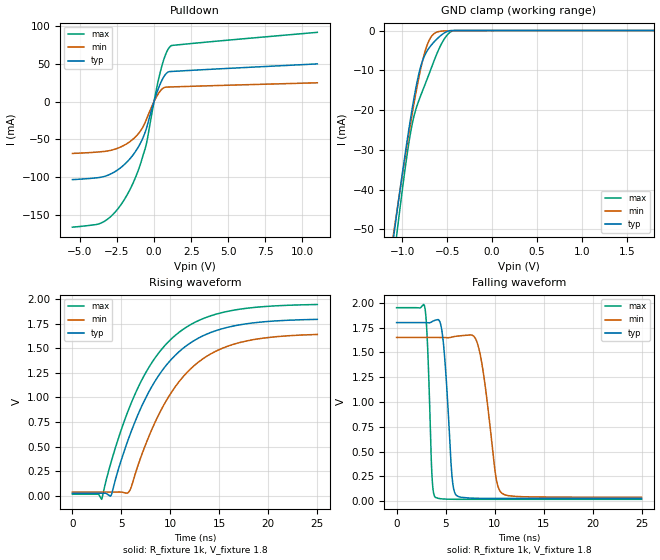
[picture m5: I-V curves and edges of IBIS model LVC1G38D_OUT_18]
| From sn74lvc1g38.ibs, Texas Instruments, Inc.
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[Model]   LVC1G38D_OUT_18
Model_type  Open_drain
Enable   Active-High
Vref =   1.8
Rref =   1000
Cref =   30p
Vmeas =   0.9
| variable   typ   min   max
C_comp   4.16pF   3.36pF   5.08pF
| C_pulldown   8.66pF   4.89pF   13.94pF
| C_tri-state   4.16pF   3.36pF   5.08pF
[Temperature Range]   40   100   -40
| Ambient temperature   25   85   -40
[Voltage range]   1.8   1.65   1.95
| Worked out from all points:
|   slope of the pulldown table from 0 to 0.27 V, typ, clamps not added: 16.8 ohm
|   GND clamp passes 1 mA (typ) near -0.56 V on its own axis
|   rising waveform, R_fixture 1k, V_fixture 1.8: 20-80 % time 5.58ns typ, 5.52ns min, 5.61ns max; typ from 0.027 V to 1.79 V
|   falling waveform, R_fixture 1k, V_fixture 1.8: 20-80 % time 650ps typ, 1.18ns min, 384ps max; typ from 1.8 V to 0.027 V
[GND Clamp]
| LVC1G38D_OUT_18
|   Voltage   I(typ)   I(min)   I(max)
-5.5V     -916.4mA   -845.5mA   -1.045A
-1.115V   -54.98mA   -53.86mA   -61.45mA
-1.085V   -49.92mA   -49.21mA   -55.72mA
-1.055V   -44.94mA   -44.63mA   -50.09mA
-910mV    -22.43mA   -23.64mA   -25.96mA
-860mV    -15.79mA   -17.12mA   -20.67mA
-795mV    -9.083mA   -9.641mA   -16.36mA
-725mV    -5.18mA    -3.758mA   -12.29mA
-670mV    -3.475mA   -1.333mA   -9.01mA
-565mV    -1.144mA   -165.1uA   -3.4mA
-475mV    -48.31uA   -65.08uA   -556uA
1.8V      20.21pA    264.6pA    784.5pA
[Pulldown]
| LVC1G38D_OUT_18
|   Voltage   I(typ)   I(min)   I(max)
-5.5V     -103.4mA   -68.72mA   -166.4mA
-3.32V    -99.02mA   -66.01mA   -158.4mA
-2.515V   -91.42mA   -62.29mA   -144mA
-1.745V   -78.46mA   -54.7mA    -121.2mA
-1.13V    -62.51mA   -44.26mA   -94.65mA
-600mV    -40.65mA   -27.77mA   -62.5mA
-450mV    -31.26mA   -20.5mA    -49.8mA
10mV      654.1uA    412.9uA    1.064mA
410mV     23.11mA    13.75mA    38.36mA
775mV     36.12mA    19.1mA     62.15mA
1.11V     39.81mA    19.36mA    73.37mA
11V       49.91mA    24.89mA    91.75mA
[Ramp]
| LVC1G38D_OUT_18
| variable   typ   min   max
dV/dt_r   1.08/5.59E-09   0.97/5.53E-09   1.19/5.63E-09
dV/dt_f   1.08/6.67E-10   0.98/1.20E-09   1.18/3.96E-10
R_load = 1k
[Rising Waveform]
| LVC1G38D_OUT_18
R_fixture =   1k
C_fixture =   0
L_fixture =   0
V_fixture =   1.8
V_fixture_min = 1.65
V_fixture_max = 1.95
|   Time   V(typ)   V(min)   V(max)
0s        27.26mV    39.51mV    18.19mV
2.63ns    27.25mV    39.51mV    18.99mV
2.99ns    27.26mV    39.5mV     -33.59mV
3.955ns   6.535mV    39.52mV    345.3mV
5.705ns   574.6mV    35.03mV    869.1mV
8.13ns    1.115V     680.4mV    1.357V
10.87ns   1.463V     1.158V     1.66V
13.19ns   1.619V     1.383V     1.794V
16ns      1.716V     1.526V     1.877V
24.99ns   1.793V     1.64V      1.944V
[Falling Waveform]
| LVC1G38D_OUT_18
R_fixture =   1k
C_fixture =   0
L_fixture =   0
V_fixture =   1.8
V_fixture_min = 1.65
V_fixture_max = 1.95
|   Time   V(typ)   V(min)   V(max)
0s        1.8V       1.65V      1.95V
2.87ns    1.8V       1.65V      1.96V
3.615ns   1.809V     1.65V      251.5mV
3.98ns    1.825V     1.65V      36.86mV
4.705ns   1.658V     1.649V     22.09mV
5.645ns   263.6mV    1.654V     18.92mV
6.12ns    56.66mV    1.663V     18.52mV
8.31ns    28.73mV    1.571V     18.2mV
10.73ns   27.4mV     81.37mV    18.19mV
24.99ns   27.26mV    39.52mV    18.19mV
